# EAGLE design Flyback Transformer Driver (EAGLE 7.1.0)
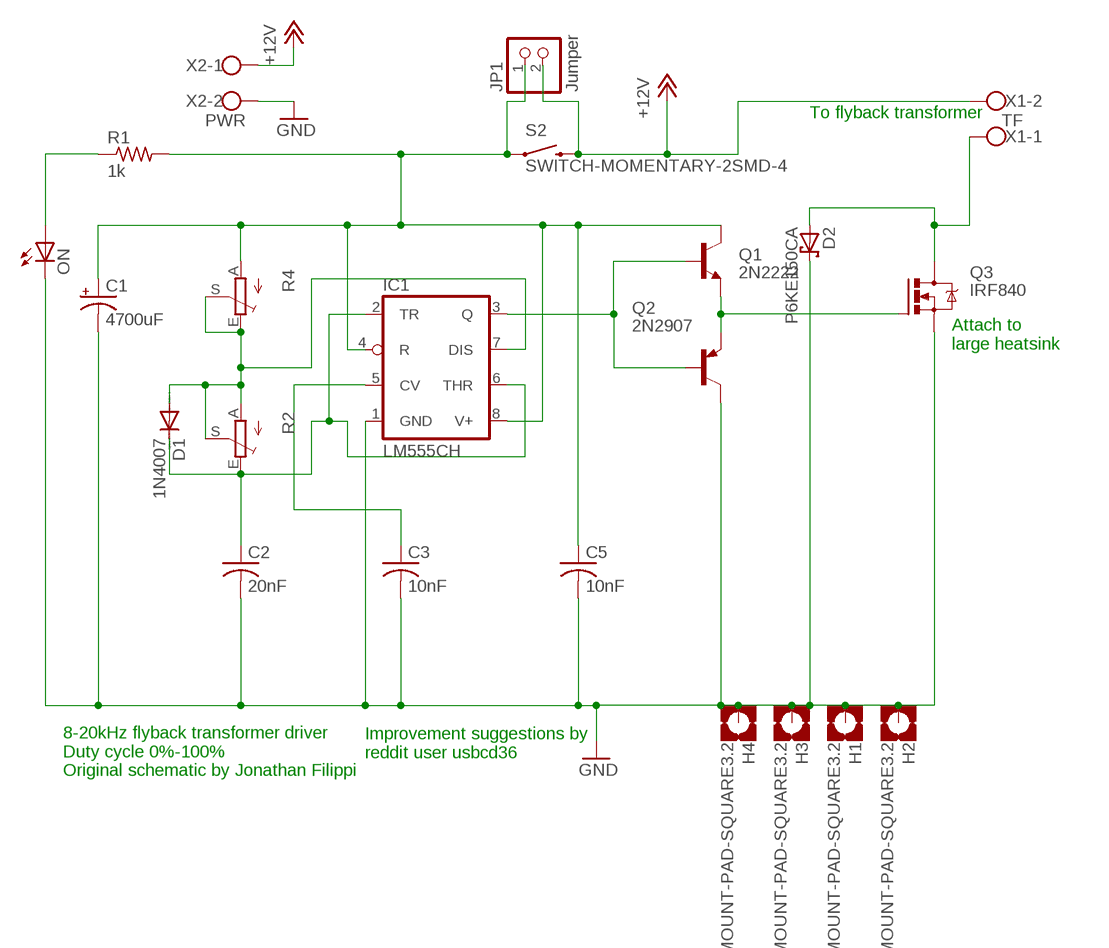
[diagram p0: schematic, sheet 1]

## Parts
C1  4700uF  CPOL-USE7.5-16  [E7,5-16]
C2  20nF  C-USC0805K  [C0805K]
C3  10nF  C-USC0805K  [C0805K]
C5  10nF  C-USC0805K  [C0805K]
D1  1N4007  DIODE-DO214AA  [DO214AA]
D2  P6KE150CA  P6KEXXA  [C1702-15]
H1  MOUNT-PAD-SQUARE3.2  [3,2-PAD-SQUARE]
H2  MOUNT-PAD-SQUARE3.2  [3,2-PAD-SQUARE]
H3  MOUNT-PAD-SQUARE3.2  [3,2-PAD-SQUARE]
H4  MOUNT-PAD-SQUARE3.2  [3,2-PAD-SQUARE]
IC1  LM555CH  LM555D  [SO08]
JP1  Jumper  PINHD-1X2  [1X02]
ON  LEDCHIPLED_1206  [CHIPLED_1206]
Q1  2N2222  TRANSISTOR_NPNMPSA42  [SOT23]
Q2  2N2907  MMBTA56-SOT23  [SOT23]
Q3  IRF840  IRF540  [TO220BV]
R1  1k  R-US_R0805  [R0805]
R2  TRIM_EU-B64W  [B64W]
R4  TRIM_EU-B64W  [B64W]
S2  SWITCH-MOMENTARY-2SMD-4  [TACTILE_SWITCH_TALL]
X1  TF  W237-102  [W237-102]
X2  PWR  W237-102  [W237-102]

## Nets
+12V: JP1.2 S2.B2 X1.2 X2.1
GND: C1.- C2.2 C3.2 C5.2 D2.C H1.B3,2(MOUNT) H2.B3,2(MOUNT) H3.B3,2(MOUNT) H4.B3,2(MOUNT) IC1.1(GND) ON.C Q2.3(C) Q3.S X2.2
N$1: C1.+ C5.1 IC1.4(R) IC1.8(V+) JP1.1 Q1.3(C) R1.2 R4.A S2.A2
N$2: ON.A R1.1
N$3: Q1.2(E) Q2.2(E) Q3.G
N$4: IC1.3(Q) Q1.1(B) Q2.1(B)
N$6: D1.A IC1.7(DIS) R2.A R2.S R4.E R4.S
N$8: C2.1 D1.C IC1.2(TR) IC1.6(THR) R2.E
N$10: C3.1 IC1.5(CV)
N$11: D2.A Q3.D X1.1

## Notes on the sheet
- To flyback transformer
- Attach to
  large heatsink
- Improvement suggestions by
  reddit user usbcd36
- 8-20kHz flyback transformer driver
  Duty cycle 0%-100%
  Original schematic by Jonathan Filippi

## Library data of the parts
C1 = rcl:CPOL-US: POLARIZED CAPACITOR, American symbol
C2 C3 C5 = rcl:C-US: CAPACITOR, American symbol
D1 = diode:DIODE-: DIODE
D2 = diode:P6KEXXA: DIODE
H1-H4 = holes:MOUNT-PAD-SQUARE: MOUNTING PAD, square
IC1 = linear:*555: TIMER
JP1 = pinhead:PINHD-1X2: PIN HEADER
ON = led:LED: LED
Q1 = SparkFun-DiscreteSemi:TRANSISTOR_NPN: Generic NPN BJT MMBT2222A - TRANS-08049 (SOT-23, 1A 40V) MPSA42 - TRANS-09116 (SOT-23, 500mA 300V) MMBT5088LT1G - TRANS-11160 (SOT-23, 50 mA 30V) BC547 - COM-08928 (TO-92 45V 100mA) (1.Collector 2.Base 3.Emitter) 2N3904 - COM-00521 (TO-92 40V 200mA) (1.Emitter 2.Base 3.Collector) P2N2222A -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; PROD_ID: TRANS-09116; VALUE: MPSA42
Q2 = transistor-pnp:*-?: PNP Transistor
Q3 = transistor-power:IRF540: HEXFET Power MOSFET
R1 = rcl:R-US_: RESISTOR, American symbol
R2 R4 = pot:TRIM_EU-: POTENTIOMETER
S2 = SparkFun-Electromechanical:SWITCH-MOMENTARY-2: Various NO switches- pushbuttons, reed, etc; PROD_ID: SWCH-11966
X1 X2 = con-wago-500:W237-102: WAGO SCREW CLAMP; MPN: 237-102; OC_FARNELL: unknown; OC_NEWARK: 70K9898

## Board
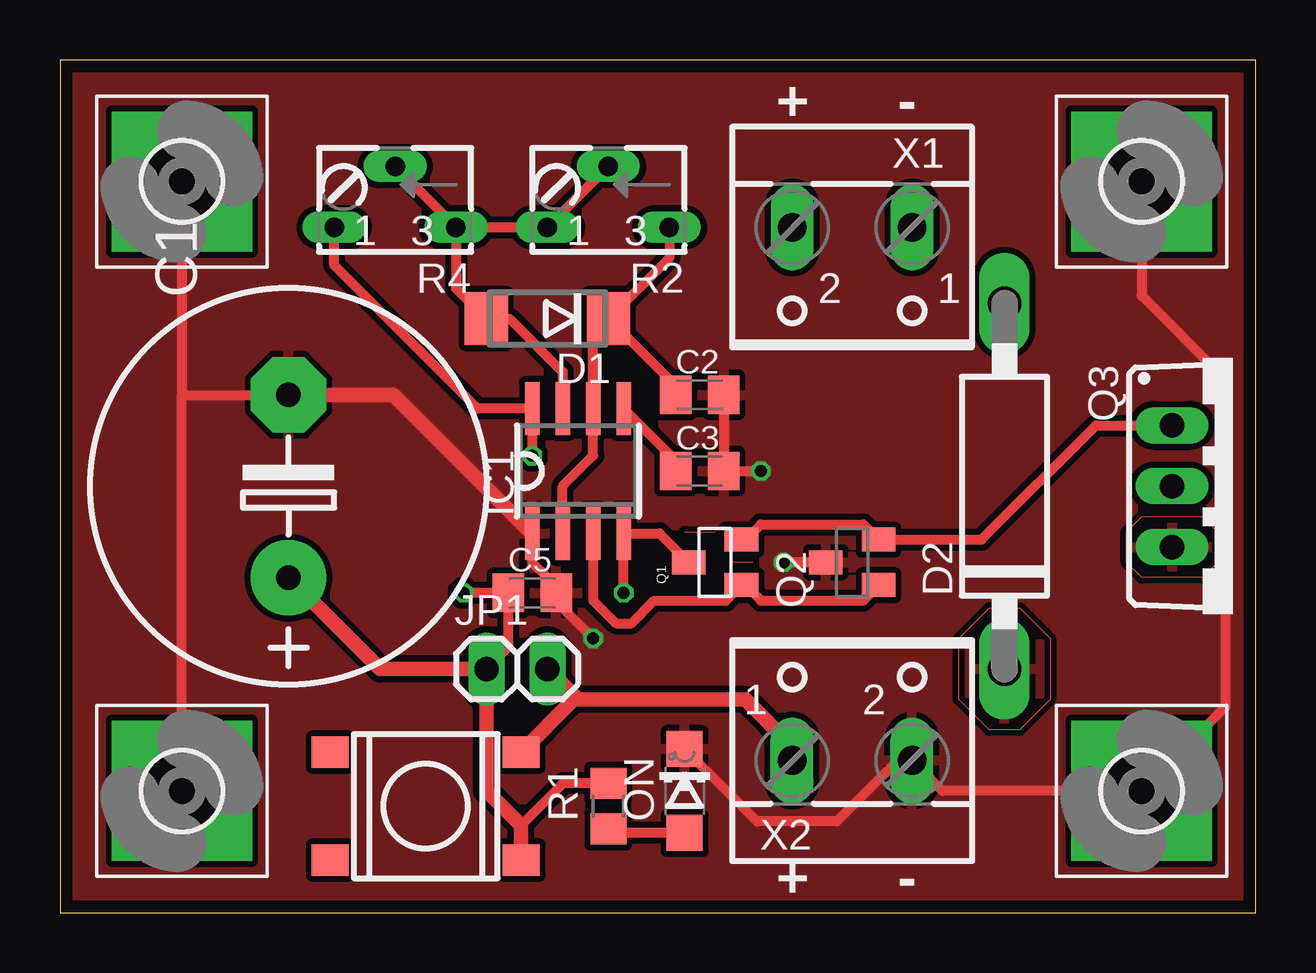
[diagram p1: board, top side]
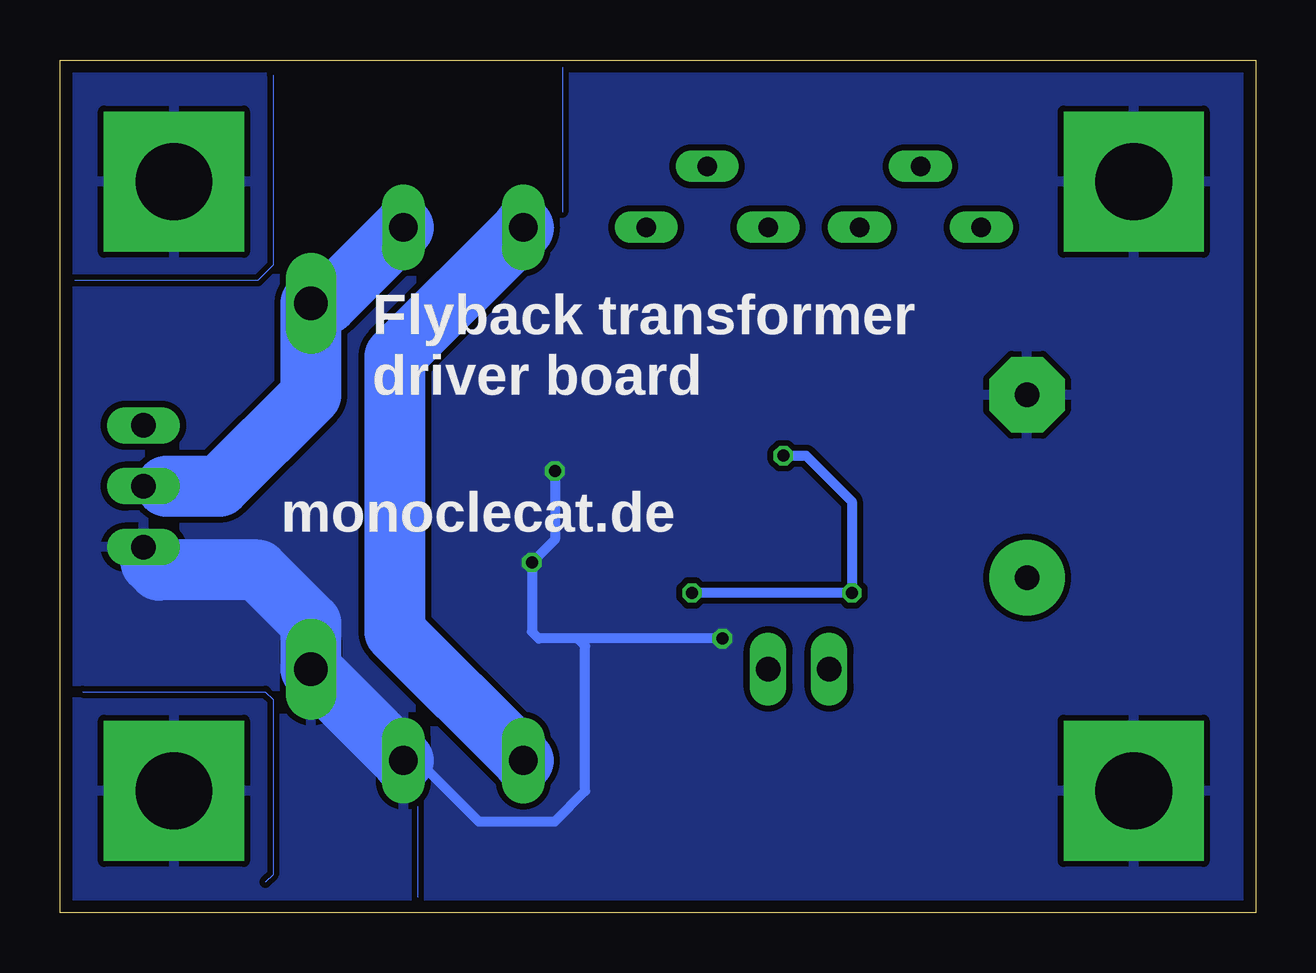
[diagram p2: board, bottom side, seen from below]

Size 49.84 x 35.55 mm. Coordinates in mm from the lower left corner, seen from the top.
Outline: 0,0 49.84,0 49.84,35.55 0,35.55 0,0
Copper layers (1*16): Top 0.035mm / dielectric 1.5mm / Bottom 0.035mm
Design rules "SmartPrototyping": minimum track width 7mil, minimum drill 12mil, track to track 7mil, track to pad 7mil, pad to pad 7mil, via to via 7mil, smd to smd 0mil, copper to edge 20mil, drill to drill 10mil, minimum pad ring 10mil, minimum via ring 6mil, stop-mask expansion 2mil, vias tented up to drill 25mil, thermal gap 10mil

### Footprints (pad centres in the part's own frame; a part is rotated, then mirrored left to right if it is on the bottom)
E7,5-16 = drill 1.016 pad 3.15: + -3.81,0 | drill 1.016 pad 3.15 octagon: - 3.81,0
C0805K = smd 1.3 x 1.6: 1 -1,0; 2 1,0
DO214AA = smd 1.8 x 2.2: A 2.55,0; C -2.55,0
C1702-15 = drill 1.397 long: A 7.62,0; C -7.62,0
3,2-PAD-SQUARE = drill 3.2 pad 5.842 square: B3,2 0,0
SO08 = smd 0.6 x 2.2: 1 -1.905,-2.6; 2 -0.635,-2.6; 3 0.635,-2.6; 4 1.905,-2.6; 5 1.905,2.6; 6 0.635,2.6; 7 -0.635,2.6; 8 -1.905,2.6
1X02 = drill 1.016 long: 1 -1.27,0; 2 1.27,0
CHIPLED_1206 = smd 1.5 x 1.5: A 0,-1.75; C 0,1.75
SOT23 = smd 1 x 1.4: 1 -0.95,-1.1; 2 0.95,-1.1; 3 0,1.1
TO220BV = drill 1.016 long: D 0,-2.54; G -2.54,-2.54; S 2.54,-2.54
R0805 = smd 1.3 x 1.5: 1 -0.95,0; 2 0.95,0
B64W = drill 0.813 long: A 2.54,0; E -2.54,0; S 0,-2.54
TACTILE_SWITCH_TALL = smd 1.55 x 1.3: A1 -3.975,-2.25; A2 3.975,-2.25; B1 -3.975,2.25; B2 3.975,2.25
W237-102 = drill 1.194 long: 1 -2.5,-1.27; 2 2.5,-1.27

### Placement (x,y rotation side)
C1  9.53,17.78 90 top
C2  26.67,21.59 0 top
C3  26.67,18.41 0 top
C5  19.68,13.34 0 top
D1  20.32,24.77 180 top
D2  39.37,17.78 90 top
H1  5.08,5.08 0 top
H2  45.09,5.08 0 top
H3  5.08,30.48 0 top
H4  45.09,30.48 0 top
IC1  21.59,18.41 0 top
JP1  19.05,10.16 0 top
ON  26.04,5.08 0 top
Q1  27.3,14.61 90 top
Q2  33.02,14.61 90 top
Q3  48.9,17.78 270 top
R1  22.86,4.45 90 top
R2  22.86,28.57 180 top
R4  13.97,28.57 180 top
S2  15.24,4.45 0 top
X1  33.02,27.3 180 top
X2  33.02,7.62 0 top

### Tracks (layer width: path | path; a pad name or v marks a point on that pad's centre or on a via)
+12V
  Top 0.61: X2.1 30.52,6.95 28.57,8.89 21.59,8.89 | 21.59,8.89 JP1.2 | 21.59,8.89 21.41,8.89 S2.B2
  Bottom 2.54: X1.2 30.52,28.54 35.88,23.18 35.88,11.71 X2.1
GND  (via drill 0.5 pad 0.41)
  Top 0.406: IC1.1 19.68,14.61 20.32,13.97 20.32,13.7 C5.2 20.68,12.97 v22.23,11.43 | ON.C 29.05,3.81 32.38,3.81 34.92,6.35 X2.2 36.79,5.08 H2.B3,2 48.58,8.57 48.58,22.23 45.09,25.72 H4.B3,2 | Q2.3 v30.16,14.61 | C2.2 C3.2 v29.21,18.41 | H3.B3,2 5.08,21.59 | H1.B3,2 5.08,21.59 | 5.08,21.59 C1.-
  Top 0.61: C1.- 13.91,21.59 IC1.1
  Bottom 0.406: v29.21,18.41 29.21,15.56 v30.16,14.61 30.16,11.71 29.89,11.43 28.26,11.43 | v22.23,11.43 28.26,11.43 | X2.2 34.92,6.35 32.38,3.81 29.21,3.81 27.94,5.08 27.94,11.11 28.26,11.43
  Bottom 1.016: 46.04,14.61 46.04,14.92 Q3.S
  Bottom 2.54: X2.2 35.56,6.35 D2.C 39.37,12.06 41.59,14.29 45.72,14.29 46.04,14.61
  pour Bottom (isolate 0.254): 0.64,0.64 0.64,34.92 49.53,34.92 49.53,0.64
  pour Top (isolate 0.254): 0.64,34.92 49.53,34.92 49.53,0.64 0.64,0.64
N$1  (via drill 0.5 pad 0.41)
  Top 0.406: JP1.1 18.68,11.06 C5.1 v16.83,13.34 | v23.5,13.34 IC1.4 25,15.81 Q1.3 | R1.2 20.96,5.39 19.21,3.65 | v19.68,19.05 IC1.8 17.4,21.02 11.43,26.99 R4.A
  Top 0.61: S2.A2 19.21,3.65 17.78,5.08 JP1.1 13.34,10.16 C1.+
  Bottom 0.406: v23.5,13.34 v16.83,13.34 16.83,17.14 18.73,19.05 v19.68,19.05
N$2
  Top 0.406: ON.A 22.86,3.33 R1.1
N$3
  Top 0.406: Q1.2 28.57,15.55 29.21,16.19 33.48,16.19 Q2.2 38.41,15.55 43.18,20.32 Q3.G
N$4
  Top 0.406: IC1.3 22.23,13.02 23.18,12.06 23.81,12.06 24.77,13.02 27.77,13.02 Q1.1 28.57,13.65 29.21,13.02 33.48,13.02 Q2.1
N$5
  Bottom 0: 34.92,4.45 34.92,0.64
N$6
  Top 0.406: R4.S R4.E | R4.E R2.A R2.S | R4.E 16.51,26.02 D1.A 18.73,24.77 20.95,22.54 IC1.7
N$7
  Bottom 0: 28.89,35.24 28.89,29.21
N$8
  Top 0.406: IC1.2 20.95,17.78 22.23,19.05 IC1.6 22.23,24.12 D1.C | R2.E 25.4,27.3 D1.C | C2.1 25.67,21.96 D1.C
N$9
  Bottom 0: 40.96,34.92 40.96,26.99 41.59,26.35 49.21,26.35
N$10
  Top 0.406: C3.1 25.67,18.84 IC1.5
N$11
  Bottom 1.422: Q3.D 45.4,17.78
  Bottom 2.54: 45.4,17.78 43.18,17.78 39.37,21.59 D2.A 38.7,25.4 X1.1
N$12
  Bottom 0: 48.9,9.21 41.27,9.21 40.96,8.89 40.96,1.59 41.27,1.27
N$13
  Top 0: 45.09,16.51 47.62,16.51 48.26,15.88 48.26,14.61 47.62,13.97 45.09,13.97 44.45,14.61 44.45,15.88 45.09,16.51
N$14
  Top 0: 40.01,12.7 41.27,11.43 41.27,8.89 40.01,7.62 38.73,7.62 37.47,8.89 37.47,11.43 38.73,12.7 40.01,12.7
N$15
  Top 0: 28.89,14.61 27.94,14.61
N$16
  Top 0: 26.04,15.88 27.3,15.88

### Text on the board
_tsilk: + | - | + | -
_bsilk: Flyback transformer / driver board | monoclecat.de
